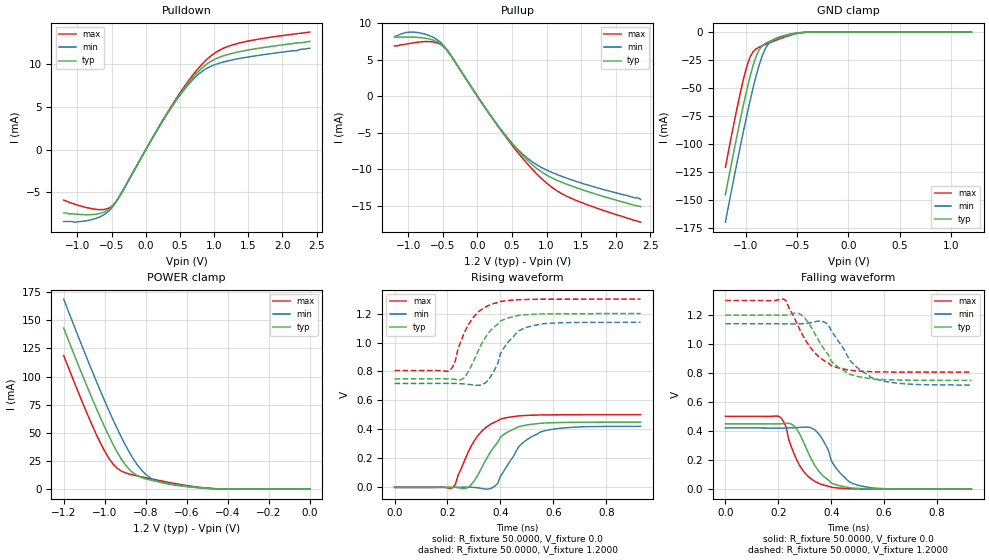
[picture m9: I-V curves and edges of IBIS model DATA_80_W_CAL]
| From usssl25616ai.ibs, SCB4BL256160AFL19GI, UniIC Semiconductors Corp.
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|   Model DATA_80_W_CAL
[Model]  DATA_80_W_CAL
Model_type I/O
Polarity   Non-Inverting
Enable   Active-High
Vinl =   0.3800V
Vinh =   0.8200V
Vmeas =  0.6000V
Cref =   5.0000pF
Rref =   50.0000
Vref =   0.6000V
C_comp   1.7430pF   1.7110pF   1.7640pF
[Temperature Range]   25.0000   85.0000   -40.0000
[Voltage Range]   1.2000V   1.1400V   1.3000V
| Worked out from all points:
|   slope of the pulldown table from 0 to 0.18 V, typ, clamps not added: 72.3 ohm
|   slope of the pullup table from 0 to 0.18 V, typ, clamps not added: 72.5 ohm
|   GND clamp passes 1 mA (typ) near -0.50 V on its own axis
|   POWER clamp passes 1 mA (typ) near -0.51 V on its own axis
|   rising waveform, R_fixture 50.0000, V_fixture 0.0: 20-80 % time 93.1ps typ, 104ps min, 93.2ps max; typ from 0 V to 0.45 V
|   rising waveform, R_fixture 50.0000, V_fixture 1.2000: 20-80 % time 87.8ps typ, 81.1ps min, 77.6ps max; typ from 0.75 V to 1.2 V
|   falling waveform, R_fixture 50.0000, V_fixture 0.0: 20-80 % time 84.5ps typ, 80.4ps min, 73.5ps max; typ from 0.45 V to 0 V
|   falling waveform, R_fixture 50.0000, V_fixture 1.2000: 20-80 % time 102ps typ, 112ps min, 103ps max; typ from 1.2 V to 0.75 V
[Pulldown]
|Voltage   I(typ)   I(min)   I(max)
-1.2V     -7.4mA     -8.4mA     -5.9mA
-1.04V    -7.53mA    -8.48mA    -6.37mA
-720mV    -7.53mA    -8.01mA    -6.977mA
-600mV    -7.269mA   -7.547mA   -6.976mA
-480mV    -6.557mA   -6.63mA    -6.508mA
-360mV    -5.125mA   -5.113mA   -5.145mA
360mV     4.827mA    4.762mA    4.915mA
640mV     8.002mA    7.795mA    8.243mA
840mV     9.703mA    9.272mA    10.17mA
1.04V     10.72mA    10.05mA    11.49mA
1.28V     11.33mA    10.55mA    12.31mA
2.4V      12.7mA     11.9mA     13.79mA
[Pullup]
|Voltage   I(typ)   I(min)   I(max)
-1.2V     8.1mA      8.2mA      6.9mA
-1.04V    8.11mA     8.74mA     7.15mA
-880mV    8.08mA     8.76mA     7.39mA
-680mV    7.819mA    8.248mA    7.489mA
-520mV    7.078mA    7.259mA    7.032mA
-400mV    5.766mA    5.835mA    5.8mA
320mV     -4.305mA   -4.323mA   -4.396mA
560mV     -7.129mA   -7.024mA   -7.403mA
760mV     -9.09mA    -8.741mA   -9.642mA
1.04V     -10.99mA   -10.26mA   -12.18mA
1.32V     -12.13mA   -11.3mA    -13.81mA
2.36V     -15.1mA    -14.1mA    -17.23mA
[GND_clamp]
|Voltage   I(typ)   I(min)   I(max)
-1.2V     -145.3mA   -169.7mA   -120.8mA
-1.11V    -103.1mA   -127.3mA   -78.51mA
-1.05V    -76.2mA    -100.1mA   -52.43mA
-990mV    -51.2mA    -74mA      -30.39mA
-960mV    -39.9mA    -61.63mA   -22.48mA
-900mV    -21.67mA   -39mA      -15mA
-870mV    -15.78mA   -29.25mA   -13.45mA
-810mV    -10.04mA   -14.72mA   -11.07mA
-750mV    -7.557mA   -7.71mA    -8.865mA
-600mV    -3.111mA   -2.463mA   -3.804mA
-420mV    -215.4uA   -156.1uA   -235uA
1.2V      1.597nA    5.589nA    1.463nA
[POWER_clamp]
|Voltage   I(typ)   I(min)   I(max)
-1.2V     143mA      168.8mA    118.7mA
-1.06V    79.88mA    104.3mA    56.26mA
-1.02V    63.08mA    86.79mA    40.63mA
-980mV    47.32mA    69.97mA    27.48mA
-940mV    33.2mA     54.05mA    18.67mA
-880mV    17.43mA    32.78mA    13.45mA
-840mV    11.87mA    21.34mA    11.69mA
-800mV    9.133mA    13.1mA     10.12mA
-720mV    6.135mA    5.731mA    7.166mA
-560mV    1.838mA    1.456mA    2.161mA
-420mV    156.9uA    132.7uA    153uA
0V        1.597nA    1.927nA    2.16nA
[Ramp]
| variable   typ   min   max
dV/dt_r  0.2701/95.9095p   0.2529/0.1060n   0.3011/86.6477p
dV/dt_f  0.2703/0.1038n   0.2535/0.1133n   0.2963/96.2373p
R_load = 50.0000
[Rising Waveform]
R_fixture= 50.0000
V_fixture= 0.0
V_fixture_min= 0.0
V_fixture_max= 0.0
|time   V(typ)   V(min)   V(max)
0s        0V         0V         0V
220ps     1.302mV    185.3uV    -1.621mV
270ps     -7.188mV   1.356mV    208.8mV
290ps     19.5mV     1.108mV    286mV
360ps     236.4mV    -9.849mV   432.3mV
390ps     310.9mV    27.48mV    459.3mV
400ps     346.6mV    75.52mV    471.2mV
470ps     419.3mV    281.9mV    493.6mV
550ps     442.3mV    381.7mV    499.9mV
930ps     450.1mV    421.5mV    501.8mV
[Rising Waveform]
R_fixture= 50.0000
V_fixture= 1.2000
V_fixture_min= 1.1400
V_fixture_max= 1.3000
|time   V(typ)   V(min)   V(max)
0s        749.5mV    717.3mV    806.2mV
210ps     748.3mV    717.8mV    807.1mV
260ps     752.1mV    714.2mV    1.05V
300ps     876.7mV    706.3mV    1.178V
340ps     1.025V     717.4mV    1.241V
380ps     1.113V     818mV      1.272V
400ps     1.148V     922.3mV    1.283V
470ps     1.187V     1.081V     1.296V
520ps     1.194V     1.115V     1.298V
930ps     1.2V       1.14V      1.3V
[Falling Waveform]
R_fixture= 50.0000
V_fixture= 0.0
V_fixture_min= 0.0
V_fixture_max= 0.0
|time   V(typ)   V(min)   V(max)
0s        450.1mV    421.6mV    501.8mV
210ps     450.5mV    421.2mV    492.6mV
230ps     452.6mV    421.2mV    425.9mV
250ps     447.6mV    422.4mV    289mV
280ps     382.1mV    425.5mV    165.7mV
330ps     188.6mV    417.5mV    63.22mV
370ps     90.71mV    334.2mV    29.11mV
420ps     29.49mV    141.4mV    9.08mV
490ps     6.533mV    33.67mV    1.919mV
930ps     748nV      5.787uV    0V
[Falling Waveform]
R_fixture= 50.0000
V_fixture= 1.2000
V_fixture_min= 1.1400
V_fixture_max= 1.3000
|time   V(typ)   V(min)   V(max)
0s        1.2V       1.14V      1.3V
220ps     1.199V     1.139V     1.31V
290ps     1.197V     1.139V     1.069V
370ps     974mV      1.154V     889.3mV
390ps     923.2mV    1.132V     867.6mV
420ps     849.8mV    1.039V     839.5mV
480ps     786mV      869.4mV    817.5mV
560ps     759.1mV    763.6mV    809mV
680ps     751.1mV    725.9mV    806.6mV
930ps     749.5mV    717.5mV    806.2mV
